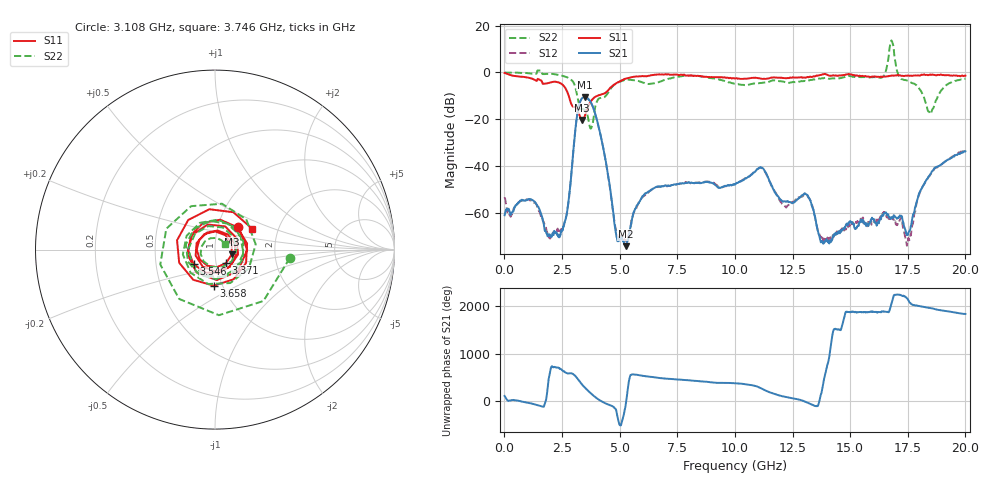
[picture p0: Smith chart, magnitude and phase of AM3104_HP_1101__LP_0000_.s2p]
!Created with skrf (http://scikit-rf.org).
# Hz S RI R 50.0
!freq ReS11 ImS11 ReS21 ImS21 ReS12 ImS12 ReS22 ImS22
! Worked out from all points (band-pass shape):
!   1601 points, 10 MHz to 20 GHz, reference 50 ohm
!   highest |S21| = -10.53 dB at 3.483 GHz (marker M1); lowest = -74.3 dB at 5.27 GHz (marker M2)
!   |S21| within 3 dB of the highest: 3.249 GHz to 3.787 GHz (538.6 MHz wide, 15.3 % of centre)
!   lowest |S11| = -20.3 dB at 3.358 GHz (marker M3), VSWR 1.21, Z = 60.2 - j3.28 ohm
!   |S11| at or under -10 dB: 2.791 GHz to 4.029 GHz (1.239 GHz wide, 36.3 % of centre)
!   |S22| runs from -24.0 to 13.7 dB; largest |S21 - S12| = 0.012
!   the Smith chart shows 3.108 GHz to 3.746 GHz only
!   S11 on the Smith chart (normalised r, x): 3.108 GHz: 1.25, +0.33; 3.371 GHz: 1.12, -0.17; 3.546 GHz: 0.78, -0.13; 3.658 GHz: 0.91, -0.38; 3.746 GHz: 1.47, +0.36
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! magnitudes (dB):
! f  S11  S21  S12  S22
! 10 MHz  -0.2  -61.1  -53.4  0.0
! 2.434 GHz  -4.7  -69.5  -67.9  -1.3
! 2.746 GHz  -8.8  -57.9  -57.6  -2.2
! 3.108 GHz  -14.8  -21.9  -21.8  -7.5
! 3.346 GHz  -20.2  -11.3  -11.4  -15.7
! 3.358 GHz  -20.3  -11.2  -11.2  -15.7
! 3.371 GHz  -20.2  -11.0  -11.1  -15.7
! 3.483 GHz  -18.8  -10.5  -10.6  -15.9
! 3.546 GHz  -16.8  -10.7  -10.7  -16.6
! 3.658 GHz  -13.9  -11.5  -11.6  -20.8
! 3.746 GHz  -12.5  -12.6  -12.7  -24.0
! 4.858 GHz  -4.6  -70.0  -67.9  -4.7
! 5.27 GHz  -2.7  -74.3  -71.8  -3.1
! 6.682 GHz  -0.8  -48.7  -48.9  -4.2
! 10.01 GHz  -2.6  -48.0  -47.8  -4.9
! 11.14 GHz  -2.7  -40.7  -40.8  -4.5
! 13.34 GHz  -1.9  -57.1  -56.6  -3.2
! 13.82 GHz  -0.8  -73.0  -71.9  -2.6
! 16.68 GHz  -1.5  -62.0  -62.7  7.2
! 17.53 GHz  -1.4  -69.0  -70.8  -3.7
! 18.45 GHz  -1.0  -43.9  -44.2  -17.2
! 20 GHz  -1.4  -33.7  -33.2  -2.7
